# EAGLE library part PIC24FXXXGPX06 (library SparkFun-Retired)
PIC24FXXXGPX06 PIC24FXXXGP106 / PIC24FXXXDA206 PIC24FJ256GP206-I/PT for IOIO Datasheet SparkFun Products IOIO-OTG - V2.2 (DEV-13613)
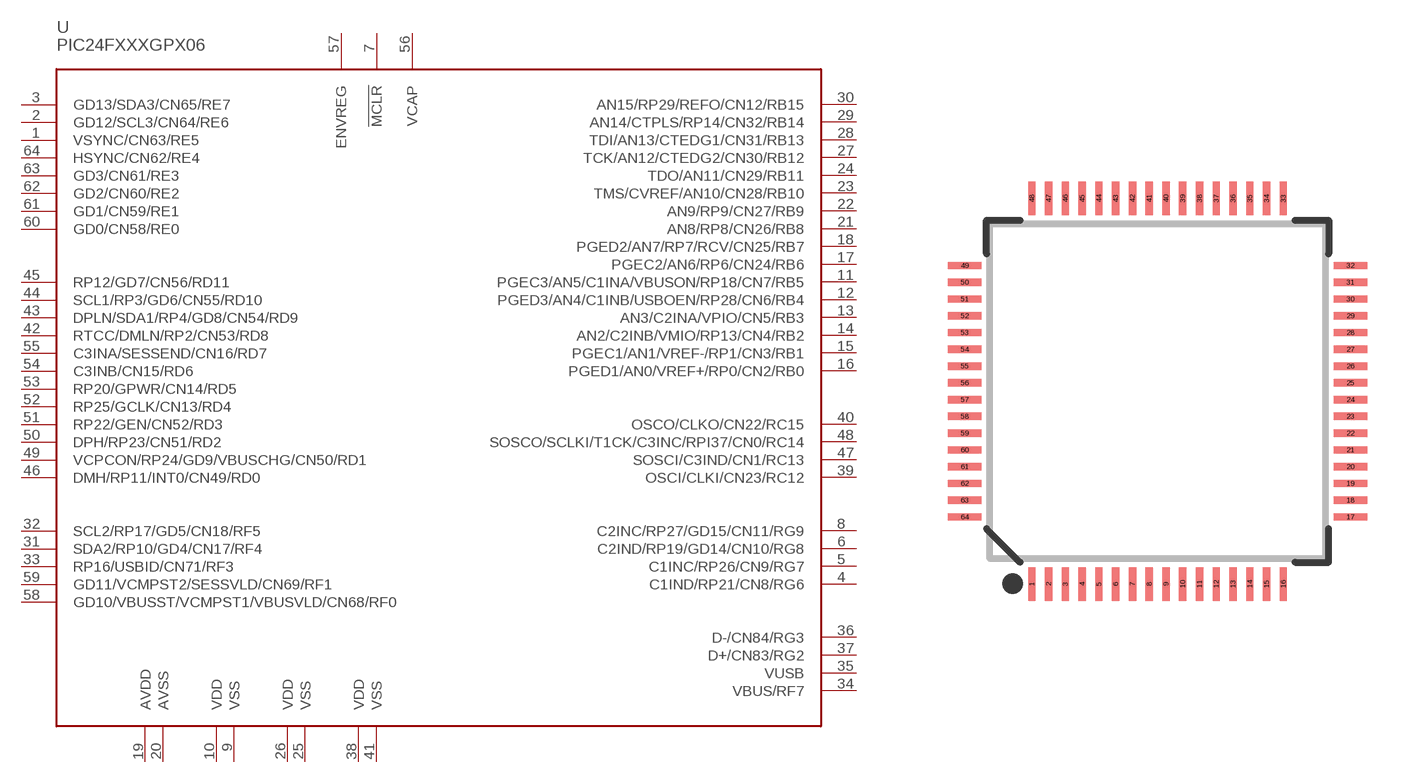
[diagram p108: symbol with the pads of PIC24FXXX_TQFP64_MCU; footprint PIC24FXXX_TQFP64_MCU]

Designator prefix U

## PIC24FXXXGPX06 (PROD_ID: IC-11312; VALUE: PIC24FJ256GB206)  [PIC24FXXX_TQFP64_MCU]
1  VSYNC/CN63/RE5
2  GD12/SCL3/CN64/RE6
3  GD13/SDA3/CN65/RE7
4  C1IND/RP21/CN8/RG6
5  C1INC/RP26/CN9/RG7
6  C2IND/RP19/GD14/CN10/RG8
7  !MCLR  in
8  C2INC/RP27/GD15/CN11/RG9
9  VSS  pwr
10  VDD  pwr
11  PGEC3/AN5/C1INA/VBUSON/RP18/CN7/RB5
12  PGED3/AN4/C1INB/USBOEN/RP28/CN6/RB4
13  AN3/C2INA/VPIO/CN5/RB3
14  AN2/C2INB/VMIO/RP13/CN4/RB2
15  PGEC1/AN1/VREF-/RP1/CN3/RB1
16  PGED1/AN0/VREF+/RP0/CN2/RB0
17  PGEC2/AN6/RP6/CN24/RB6
18  PGED2/AN7/RP7/RCV/CN25/RB7
19  AVDD  pwr
20  AVSS  pwr
21  AN8/RP8/CN26/RB8
22  AN9/RP9/CN27/RB9
23  TMS/CVREF/AN10/CN28/RB10
24  TDO/AN11/CN29/RB11
25  VSS  pwr
26  VDD  pwr
27  TCK/AN12/CTEDG2/CN30/RB12
28  TDI/AN13/CTEDG1/CN31/RB13
29  AN14/CTPLS/RP14/CN32/RB14
30  AN15/RP29/REFO/CN12/RB15
31  SDA2/RP10/GD4/CN17/RF4
32  SCL2/RP17/GD5/CN18/RF5
33  RP16/USBID/CN71/RF3
34  VBUS/RF7  in
35  VUSB  pwr
36  D-/CN84/RG3
37  D+/CN83/RG2
38  VDD  pwr
39  OSCI/CLKI/CN23/RC12
40  OSCO/CLKO/CN22/RC15
41  VSS  pwr
42  RTCC/DMLN/RP2/CN53/RD8
43  DPLN/SDA1/RP4/GD8/CN54/RD9
44  SCL1/RP3/GD6/CN55/RD10
45  RP12/GD7/CN56/RD11
46  DMH/RP11/INT0/CN49/RD0
47  SOSCI/C3IND/CN1/RC13
48  SOSCO/SCLKI/T1CK/C3INC/RPI37/CN0/RC14
49  VCPCON/RP24/GD9/VBUSCHG/CN50/RD1
50  DPH/RP23/CN51/RD2
51  RP22/GEN/CN52/RD3
52  RP25/GCLK/CN13/RD4
53  RP20/GPWR/CN14/RD5
54  C3INB/CN15/RD6
55  C3INA/SESSEND/CN16/RD7
56  VCAP  pwr
57  ENVREG  in
58  GD10/VBUSST/VCMPST1/VBUSVLD/CN68/RF0
59  GD11/VCMPST2/SESSVLD/CN69/RF1
60  GD0/CN58/RE0
61  GD1/CN59/RE1
62  GD2/CN60/RE2
63  GD3/CN61/RE3
64  HSYNC/CN62/RE4

## Footprint PIC24FXXX_TQFP64_MCU (pad centres in mm)
64-Lead TQFP Plastic Thin Quad Flatpack - 10x10x1mm Body, 2mmFP
smd 0.22 x 1: 1 -3.75,-5.75; 2 -3.25,-5.75; 3 -2.75,-5.75; 4 -2.25,-5.75; 5 -1.75,-5.75; 6 -1.25,-5.75; 7 -0.75,-5.75; 8 -0.25,-5.75; 9 0.25,-5.75; 10 0.75,-5.75; 11 1.25,-5.75; 12 1.75,-5.75; 13 2.25,-5.75; 14 2.75,-5.75; 15 3.25,-5.75; 16 3.75,-5.75; 33 3.75,5.75; 34 3.25,5.75; 35 2.75,5.75; 36 2.25,5.75; 37 1.75,5.75; 38 1.25,5.75; 39 0.75,5.75; 40 0.25,5.75; 41 -0.25,5.75; 42 -0.75,5.75; 43 -1.25,5.75; 44 -1.75,5.75; 45 -2.25,5.75; 46 -2.75,5.75; 47 -3.25,5.75; 48 -3.75,5.75
smd 1 x 0.22: 17 5.75,-3.75; 18 5.75,-3.25; 19 5.75,-2.75; 20 5.75,-2.25; 21 5.75,-1.75; 22 5.75,-1.25; 23 5.75,-0.75; 24 5.75,-0.25; 25 5.75,0.25; 26 5.75,0.75; 27 5.75,1.25; 28 5.75,1.75; 29 5.75,2.25; 30 5.75,2.75; 31 5.75,3.25; 32 5.75,3.75; 49 -5.75,3.75; 50 -5.75,3.25; 51 -5.75,2.75; 52 -5.75,2.25; 53 -5.75,1.75; 54 -5.75,1.25; 55 -5.75,0.75; 56 -5.75,0.25; 57 -5.75,-0.25; 58 -5.75,-0.75; 59 -5.75,-1.25; 60 -5.75,-1.75; 61 -5.75,-2.25; 62 -5.75,-2.75; 63 -5.75,-3.25; 64 -5.75,-3.75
